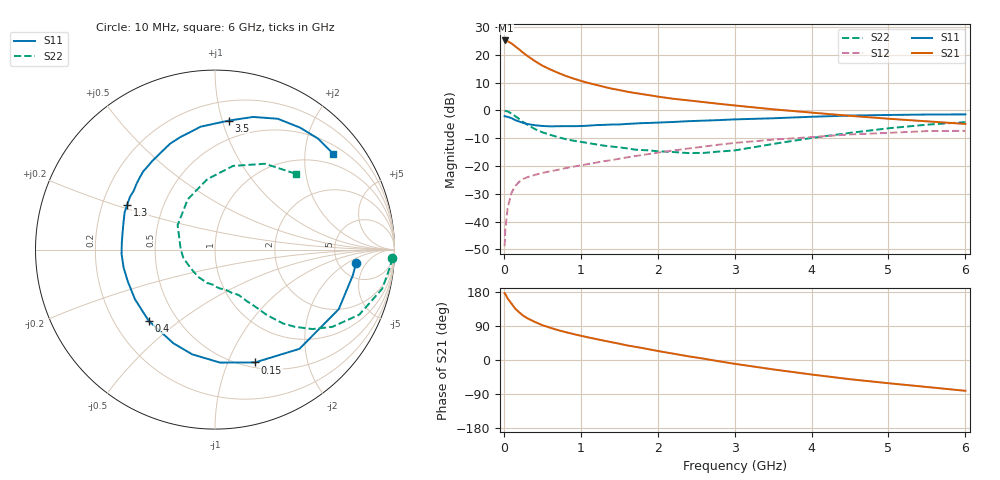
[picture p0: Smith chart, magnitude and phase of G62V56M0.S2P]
! SIEMENS Small Signal Semiconductors
! BFG193
! Si NPN RF Bipolar Junction Transistor in SOT223
! VCE = 2.5 V  IC = 6 mA
! Common Emitter S-Parameters:  August  1996
# GHz  S  MA  R  50
!  f  S11  S21  S12  S22
! GHz  MAG  ANG  MAG  ANG  MAG  ANG  MAG  ANG
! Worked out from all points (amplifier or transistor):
!   36 points, 10 MHz to 6 GHz, reference 50 ohm
!   highest |S21| = 25.2 dB at 20 MHz (marker M1)
!   |S21| within 3 dB of that: start of sweep to 188.6 MHz
!   unconditionally stable (mu >= 1): 1.022 GHz to 2.609 GHz
!   at 250 MHz: K = 0.39, MSG = 22.8 dB, |S12| = -24.7 dB
!   at 1.4 GHz: K = 1.08, MAG = 11.2 dB, |S12| = -17.9 dB
!   at 6 GHz: K = 0.89, MSG = 1.2 dB, |S12| = -7.3 dB
!   S11 on the Smith chart (normalised r, x): 10 MHz: 7.39, -2.87; 150 MHz: 0.56, -1.26; 400 MHz: 0.35, -0.39; 1.3 GHz: 0.31, +0.22; 3.5 GHz: 0.35, +1.05; 6 GHz: 0.70, +2.66
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0.01  0.7899 -5.3  18.07 176.3  0.0036 87.3  0.9881 -2.7
0.02  0.7815 -10.5  18.18 173.7  0.0074 87.0  0.9811 -5.4
0.05  0.7652 -25.7  17.57 162.3  0.0178 76.7  0.9568 -13.2
0.1  0.7261 -49.6  16.08 148.6  0.033 67.4  0.8815 -24.3
0.15  0.667 -70.5  14.18 135.0  0.0438 57.8  0.7833 -33.3
0.2  0.63 -87.5  12.51 125.7  0.0521 52.5  0.7006 -39.2
0.25  0.5972 -102.3  10.97 117.2  0.058 47.9  0.6192 -44.0
0.3  0.5708 -114.1  9.714 110.7  0.0624 45.4  0.5606 -47.3
0.4  0.5419 -133.1  7.797 100.7  0.0689 42.1  0.4655 -51.6
0.5  0.5248 -148.1  6.412 92.0  0.0747 40.4  0.4043 -54.0
0.6  0.5173 -159.8  5.492 85.3  0.0803 40.4  0.364 -56.3
0.7  0.5191 -169.0  4.783 79.1  0.0851 40.3  0.3319 -58.7
0.9  0.5206 175.7  3.768 68.7  0.0972 40.5  0.2861 -62.4
1.1  0.5315 163.6  3.118 59.6  0.1086 40.7  0.2582 -68.8
1.3  0.5491 153.2  2.663 51.1  0.1218 40.2  0.2323 -74.9
1.6  0.5714 139.7  2.178 38.6  0.1428 38.2  0.2078 -87.9
2.2  0.6195 119.0  1.624 16.8  0.1899 31.3  0.1786 -121.7
2.8  0.6701 101.6  1.314 -3.5  0.2424 21.2  0.1821 -165.4
3.5  0.7225 84.0  1.047 -24.8  0.2977 5.8  0.249 146.8
4.5  0.8084 64.4  0.8 -50.7  0.3698 -14.4  0.3943 96.3
5.5  0.8435 47.3  0.636 -71.2  0.4243 -39.3  0.5538 59.7
6  0.8482 39.0  0.571 -81.3  0.4297 -53.5  0.6163 43.3
